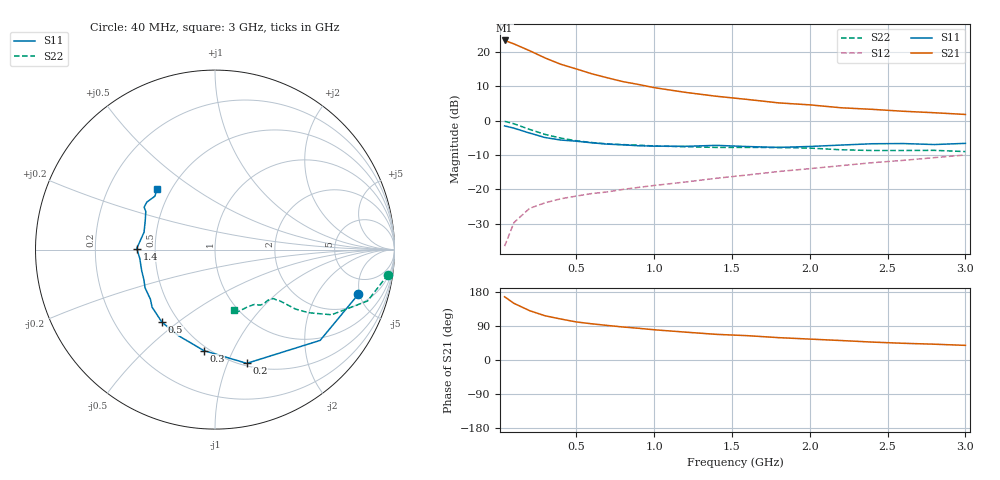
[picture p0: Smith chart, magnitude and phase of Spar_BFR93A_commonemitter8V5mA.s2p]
! Filename:  BFR93AE.S2P  Version:  2.0
! NXP part #: BFR93A  Date: May 1990
! Bias condition: Vce=8V, Ic=5mA
#  MHz  S  MA  R  50
! Freq  S11  S21  S12  S22  !GUM [dB]
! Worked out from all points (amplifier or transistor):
!   21 points, 40 MHz to 3 GHz, reference 50 ohm
!   highest |S21| = 23.2 dB at 40 MHz (marker M1)
!   |S21| within 3 dB of that: start of sweep to 201.7 MHz
!   unconditionally stable (mu >= 1): 1.095 GHz to 2.356 GHz
!   at 300 MHz: K = 0.48, MSG = 21.0 dB, |S12| = -23.9 dB
!   at 1 GHz: K = 0.98, MSG = 14.2 dB, |S12| = -18.9 dB
!   at 3 GHz: K = 0.96, MSG = 5.9 dB, |S12| = -10.0 dB
!   S11 on the Smith chart (normalised r, x): 40 MHz: 2.91, -4.84; 200 MHz: 0.53, -1.17; 300 MHz: 0.47, -0.78; 500 MHz: 0.41, -0.44; 1.4 GHz: 0.39, +0.01; 3 GHz: 0.42, +0.36
40  0.836 -17.4  14.52 166.8  0.015 80.3  0.974 -8.2
100  0.774 -40.8  12.94 149.5  0.033 69.0  0.897 -18.6
200  0.658 -74.4  10.32 130.3  0.053 58.2  0.744 -29.2
300  0.566 -96.3  8.091 116.7  0.064 52.8  0.629 -34.0
400  0.521 -113.0  6.567 108.2  0.073 50.6  0.556 -36.5
500  0.501 -126.2  5.611 100.5  0.08 51.2  0.508 -37.3
600  0.475 -137.6  4.769 95.5  0.087 52.4  0.479 -37.9
700  0.454 -142.4  4.169 91.2  0.092 53.8  0.458 -38.4
800  0.444 -151.4  3.669 87.1  0.1 56.2  0.447 -38.8
900  0.43 -157.2  3.337 83.7  0.107 57.8  0.439 -39.5
1000  0.425 -164.0  3.003 79.8  0.114 58.9  0.427 -39.8
1200  0.422 -173.4  2.565 73.6  0.128 61.8  0.416 -41.5
1400  0.436 179.2  2.25 67.7  0.145 63.8  0.407 -44.3
1600  0.419 173.0  2.022 64.2  0.162 66.4  0.407 -46.5
1800  0.407 166.3  1.803 59.0  0.182 67.1  0.405 -48.8
2000  0.42 157.8  1.688 55.2  0.2 68.0  0.398 -51.0
2200  0.44 151.2  1.532 51.4  0.221 69.1  0.376 -54.4
2400  0.46 149.1  1.453 47.3  0.244 68.8  0.367 -60.2
2600  0.463 145.2  1.363 44.1  0.264 68.2  0.367 -65.6
2800  0.448 138.4  1.297 41.7  0.289 68.0  0.369 -69.2
3000  0.466 134.0  1.225 38.6  0.316 67.2  0.354 -72.7
